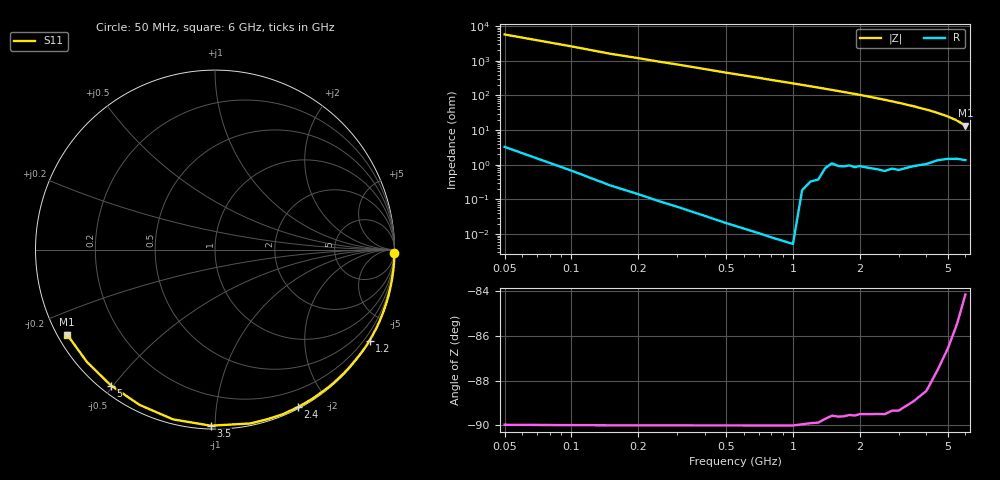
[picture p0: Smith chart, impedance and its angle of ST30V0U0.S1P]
! SIEMENS Discrete & RF Semiconductors
! BA892
! Si PIN Diode in SCD-80
! VR = 30 V
! S-Parameters:  September  1997
# GHz  S  MA  R  50
!  f  S11
! GHz  MAG  ANG
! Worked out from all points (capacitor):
!   34 points, 50 MHz to 6 GHz, reference 50 ohm
!   read as one part to ground: C = 611 fF near 50 MHz
!   lowest |Z| = 13.4 ohm at 6 GHz (marker M1)
!   S11 on the Smith chart (normalised r, x): 50 MHz: open; 1.2 GHz: 0.01, -3.67; 2.4 GHz: 0.01, -1.66; 3.5 GHz: 0.02, -0.98; 5 GHz: 0.03, -0.49; 6 GHz: 0.03, -0.27
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0.05  1 -1.0
0.15  1 -3.6
0.2  1 -4.8
0.4  1 -9.9
0.5  1 -12.6
0.6  1 -15.1
0.7  1 -17.6
0.8  1 -20.3
1  1 -25.3
1.2  0.9991 -30.5
1.3  0.9988 -33.0
1.4  0.997 -35.7
1.5  0.9953 -38.2
1.6  0.9955 -40.9
1.7  0.9951 -43.5
1.9  0.9942 -48.7
2  0.9931 -51.4
2.2  0.9927 -56.8
2.4  0.9921 -62.2
2.6  0.9919 -67.6
2.8  0.989 -73.1
3  0.9887 -78.4
3.5  0.9814 -91.4
4  0.9743 -103.9
4.5  0.9618 -115.9
5  0.9535 -127.4
5.5  0.9492 -138.7
6  0.9504 -150.1
